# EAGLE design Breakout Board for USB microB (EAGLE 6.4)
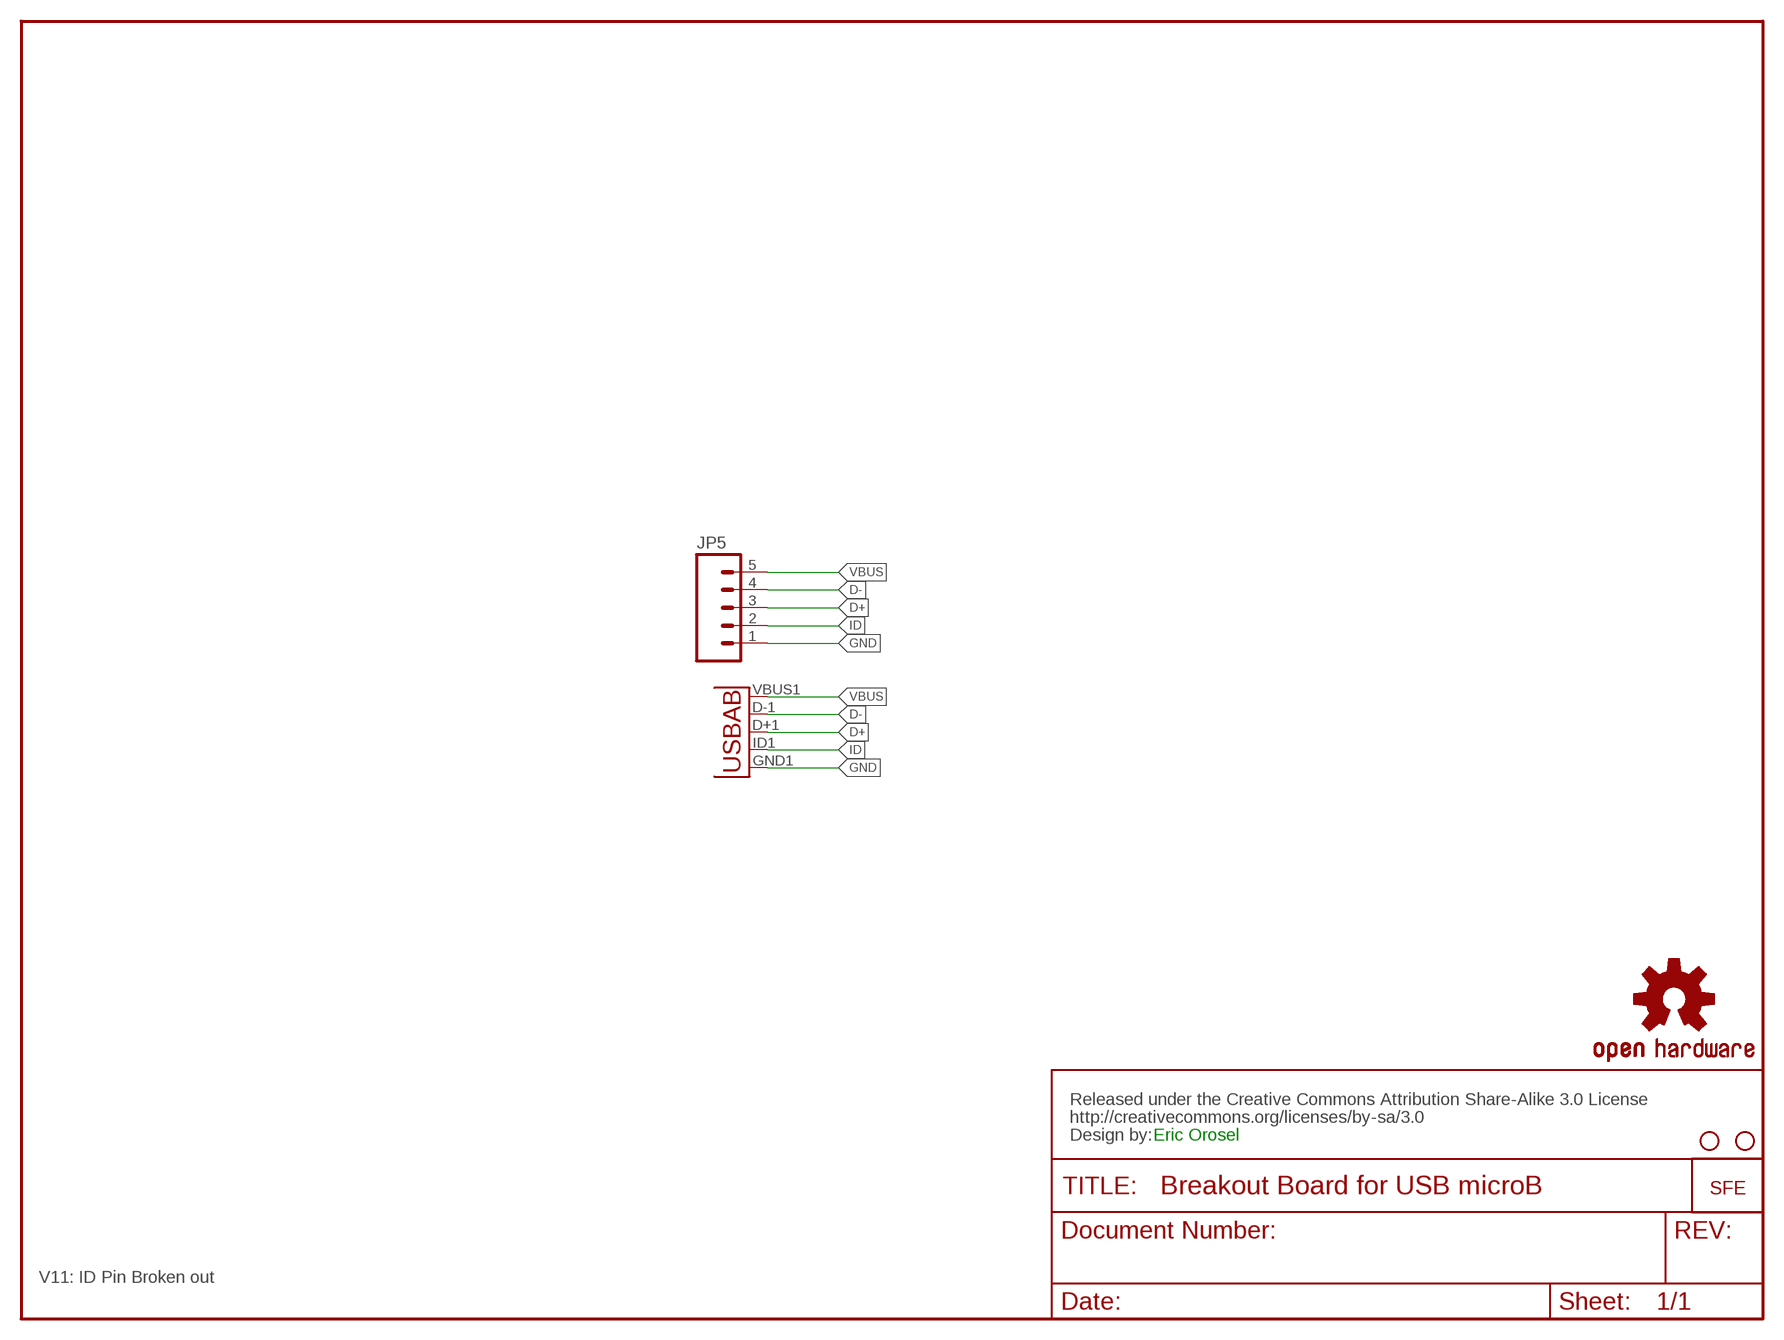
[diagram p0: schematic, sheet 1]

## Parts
JP2  LOGO-SFESK  [SFE-LOGO-FLAME]
JP3  STAND-OFF  [STAND-OFF]
JP4  STAND-OFF  [STAND-OFF]
JP5  M05PTH  [1X05]
U$2  CREATIVE_COMMONS  [CREATIVE_COMMONS]
U$3  OSHW-LOGOS  [OSHW-LOGO-S]
U$4  USB-AB""  [USB-AB-MICRO-SMD_V02_BOSS]

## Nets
D+: JP5.3 U$4.D+1(D+)
D-: JP5.4 U$4.D-1(D-)
GND: JP5.1 U$4.GND1(GND)
ID: JP5.2 U$4.ID1(USBID)
VBUS: JP5.5 U$4.VBUS1(VBUS)

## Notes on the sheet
- Eric Orosel
- V11: ID Pin Broken out

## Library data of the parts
JP2 = SparkFun:LOGO-SFE: Spark Fun Electronics PCB Logo
JP3 JP4 = SparkFun:STAND-OFF: Stand Off
JP5 = SparkFun:M05: Header 5 Standard 5-pin 0.1" header. Use with straight break away headers (SKU : PRT-00116), right angle break away headers (PRT-00553), swiss pins (PRT-00743), machine pins (PRT-00117), and female headers (PRT-00115). Molex polarized connector foot print use with SKU : PRT-08230 with associated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
U$2 = SparkFun-Aesthetics:CREATIVE_COMMONS: Creative Commons License summary
U$3 = SparkFun-Aesthetics:OSHW-LOGO: Open Source Hardware Logo This logo indicates the piece of hardware it is found on incorporates a OSHW license and/or adheres to the definition of open source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
U$4 = Testing:USB-AB: This is a USB AB connector that is compatible with USB OTG. i.e. this connector can serve as a host or device

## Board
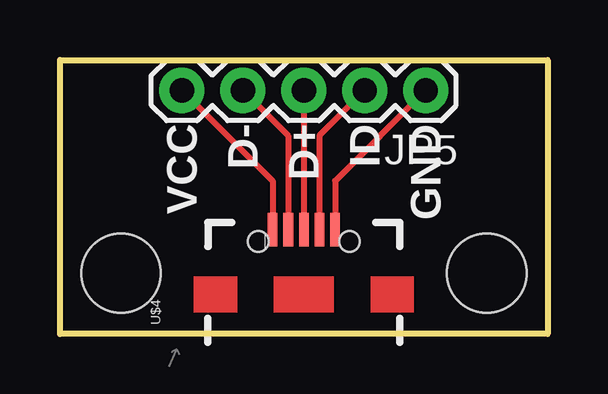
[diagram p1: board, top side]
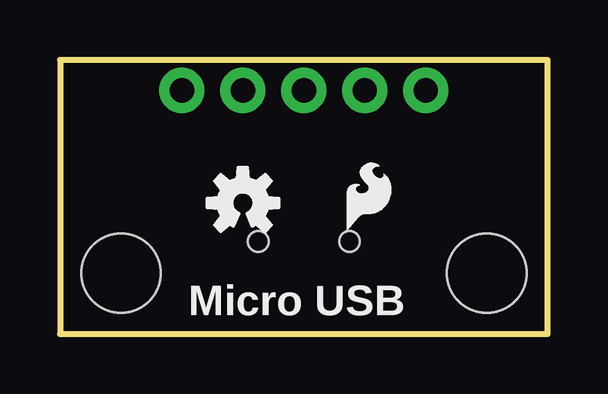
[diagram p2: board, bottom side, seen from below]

Size 20.32 x 11.43 mm. Coordinates in mm from the lower left corner, seen from the top.
Outline: 0,0 0,11.43 20.32,11.43 20.32,0 0,0
Copper layers (1*16): Top 0.035mm / dielectric 1.5mm / Bottom 0.035mm
Design rules "default": minimum track width 8mil, minimum drill 20mil, track to track 8mil, track to pad 8mil, pad to pad 8mil, via to via 8mil, smd to smd 8mil, copper to edge 9mil, drill to drill 8mil, minimum pad ring 12mil, minimum via ring 10mil, stop-mask expansion 4mil, vias tented up to drill 20mil, thermal gap 10mil

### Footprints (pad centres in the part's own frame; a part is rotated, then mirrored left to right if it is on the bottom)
STAND-OFF = hole 3.302: 0,0
1X05 = drill 1.016 pad 1.88: 1 0,0; 2 2.54,0; 3 5.08,0; 4 7.62,0; 5 10.16,0
USB-AB-MICRO-SMD_V02_BOSS = smd 1.4 x 0.4: D+1 2.7,0; D-1 2.7,0.65; GND1 2.7,-1.3; ID1 2.7,-0.65; VBUS1 2.7,1.3 | hole 0.85: 2.2,1.9; 2.2,-1.9

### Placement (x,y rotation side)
JP2  8.38,4.32 0 bottom
JP3  17.78,2.54 0 top
JP4  2.54,2.54 0 top
JP5  15.24,10.16 180 top
U$2  not placed on the board
U$3  12.7,5.46 0 bottom
U$4  10.16,1.65 90 top

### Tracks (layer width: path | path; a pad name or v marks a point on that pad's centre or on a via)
D+
  Top 0.254: JP5.3 U$4.D+1
D-
  Top 0.254: JP5.4 9.51,8.27 U$4.D-1
GND
  Top 0.254: JP5.1 11.46,6.38 U$4.GND1
ID
  Top 0.254: JP5.2 10.81,8.27 U$4.ID1
VBUS
  Top 0.254: JP5.5 8.86,6.38 U$4.VBUS1

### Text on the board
tPlace: VCC | D- | D+ | ID | GND
bPlace: Micro USB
